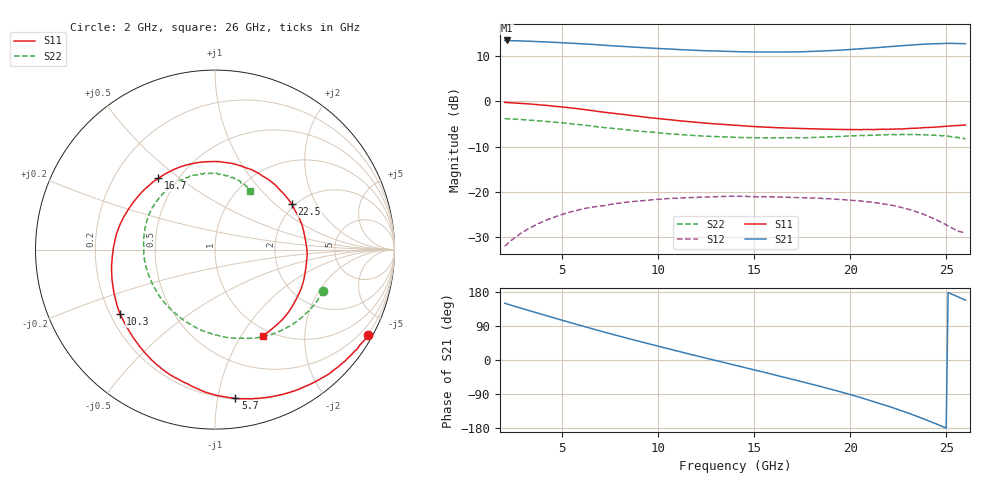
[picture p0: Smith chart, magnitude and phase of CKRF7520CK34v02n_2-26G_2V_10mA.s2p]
! CHUO DENSHI KOGYO Co.,Ltd.
! 29. March 2016
! CKRF7520CK34
! N-channel HJ-FET
! Vds = 2 V Id = 10 mA
# Hz S  MA  R 50
!  f  S11  S21  S12  S22
!  Hz  MAG  ANG  MAG  ANG  MAG  ANG  MAG  ANG
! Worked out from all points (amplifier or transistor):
!   241 points, 2 GHz to 26 GHz, reference 50 ohm
!   highest |S21| = 13.5 dB at 2.1 GHz (marker M1)
!   |S21| within 3 dB of that: start of sweep to end of sweep
!   unconditionally stable (mu >= 1): 14.17 GHz to end of sweep
!   at 6 GHz: K = 0.55, MSG = 18.3 dB, |S12| = -23.9 dB
!   at 14 GHz: K = 0.99, MSG = 16.0 dB, |S12| = -21.0 dB
!   at 26 GHz: K = 1.84, MAG = 15.6 dB, |S12| = -29.0 dB
!   lowest NFmin = 0.51 dB at 18 GHz
!   S11 on the Smith chart (normalised r, x): 2 GHz: 0.19, -3.85; 5.7 GHz: 0.20, -1.13; 10.3 GHz: 0.24, -0.29; 16.7 GHz: 0.39, +0.42; 22.5 GHz: 1.93, +1.29; 26 GHz: 0.91, -1.25
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2e9  0.9758 -29.1  4.733 149.8  0.02499 69.6  0.6467 -21.0
2.1e9  0.9752 -30.5  4.736 148.2  0.02589 68.4  0.6423 -22.2
3.1e9  0.944 -44.8  4.658 133.0  0.03738 58.4  0.6255 -32.4
4e9  0.91 -57.7  4.575 119.5  0.04684 49.3  0.6053 -41.8
5.7e9  0.8364 -82.2  4.396 94.7  0.06192 33.0  0.5593 -59.1
6e9  0.8216 -86.4  4.362 90.4  0.06406 30.4  0.5507 -62.1
8.1e9  0.7211 -115.7  4.076 61.3  0.07569 12.6  0.492 -83.1
1e10  0.6478 -141.5  3.859 36.5  0.08225 -1.9  0.4521 -102.2
1.03e10  0.6395 -145.8  3.837 32.5  0.08368 -4.1  0.4437 -105.3
1.2e10  0.5874 -168.8  3.679 11.0  0.08685 -16.0  0.4169 -122.5
1.4e10  0.5466 164.4  3.566 -13.8  0.0894 -29.6  0.4008 -142.9
1.54e10  0.5215 145.9  3.529 -31.0  0.08841 -38.8  0.3952 -157.4
1.67e10  0.5076 128.4  3.529 -47.3  0.08699 -47.2  0.3973 -171.0
1.8e10  0.4978 110.2  3.584 -63.7  0.0854 -55.8  0.3984 175.4
2.02e10  0.4884 75.5  3.783 -94.1  0.0799 -72.4  0.4159 150.5
2.12e10  0.4882 57.2  3.916 -109.3  0.07618 -81.7  0.4222 138.1
2.2e10  0.4916 41.1  4.035 -122.3  0.07175 -90.3  0.4311 127.0
2.25e10  0.4969 30.5  4.111 -130.8  0.06836 -96.6  0.4324 119.6
2.35e10  0.506 7.1  4.262 -149.0  0.05943 -112.2  0.429 103.9
2.45e10  0.5226 -18.7  4.37 -169.0  0.0487 -133.4  0.4188 86.9
2.53e10  0.538 -40.9  4.401 173.8  0.03978 -160.6  0.4066 72.8
2.6e10  0.5494 -61.0  4.361 158.0  0.03529 165.6  0.382 59.0
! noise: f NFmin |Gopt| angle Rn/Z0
1.8e+10  0.51  0.469  -134  0.05574
1.85e+10  0.53  0.457  -127.2  0.06318
1.9e+10  0.55  0.445  -119  0.0707
2e+10  0.58  0.415  -106.3  0.08994
2.05e+10  0.6  0.391  -98.11  0.1022
2.1e+10  0.63  0.369  -93.44  0.1092
2.2e+10  0.7  0.328  -80.81  0.1189
2.25e+10  0.73  0.303  -74.04  0.1287
2.3e+10  0.76  0.277  -64.71  0.1399
2.4e+10  0.8  0.213  -50.86  0.1572
